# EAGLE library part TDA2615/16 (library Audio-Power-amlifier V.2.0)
2 ´ 6 W hi-fi audio power amplifier Philips Semiconductors
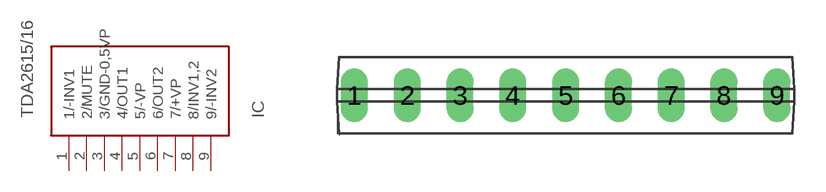
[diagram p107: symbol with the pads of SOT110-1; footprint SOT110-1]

Designator prefix IC

## TDA2615/16  [SOT110-1]
1  1/-INV1  in
2  2/MUTE  in
3  3/GND-0,5VP  pwr
4  4/OUT1  out
5  5/-VP  pwr
6  6/OUT2  out
7  7/+VP  pwr
8  8/INV1,2  in
9  9/-INV2  in

## Footprint SOT110-1 (pad centres in mm)
SIL9MPF: plastic single in-line medium power package with fin; 9 leads
drill 0.8 long: 1 -10.16,0; 2 -7.62,0; 3 -5.08,0; 4 -2.54,0; 5 0,0; 6 2.54,0; 7 5.08,0; 8 7.62,0; 9 10.16,0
